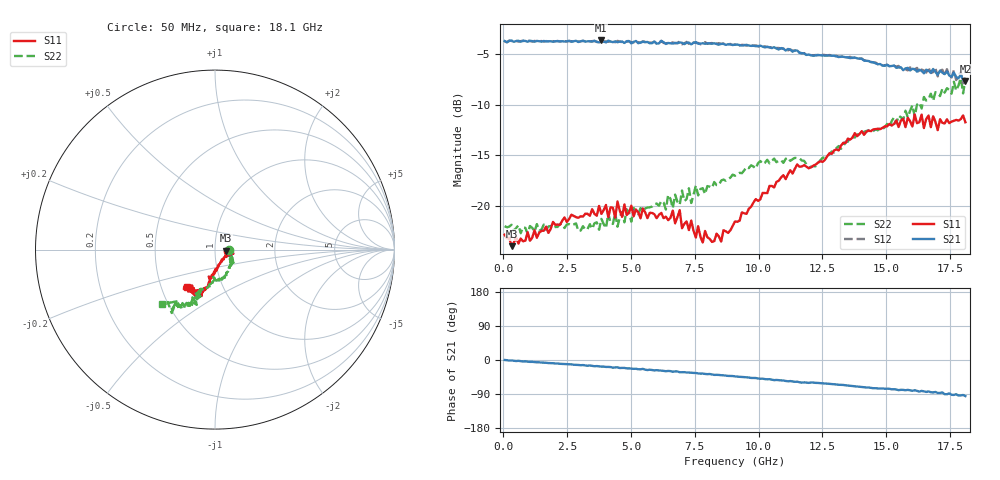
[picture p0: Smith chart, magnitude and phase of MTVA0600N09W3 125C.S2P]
! Network Analyzer HP8720D.06.14 Serial No. US36140669
! 10 May 2005  15:08:20
! Frequency  S11  S21  S12  S22
# HZ  S  DB R 50
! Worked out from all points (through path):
!   201 points, 50 MHz to 18.1 GHz, reference 50 ohm
!   highest |S21| = -3.67 dB at 3.841 GHz (marker M1); lowest = -7.7 dB at 18.1 GHz (marker M2)
!   group delay of S21, straight-line fit = 14.5 ps
!   lowest |S11| = -23.9 dB at 320.8 MHz (marker M3), VSWR 1.14, Z = 56.7 - j0.663 ohm
!   |S11| at or under -10 dB: start of sweep to end of sweep
!   |S22| runs from -22.7 to -7.4 dB; largest |S21 - S12| = 0.028
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5e7  -22.81 -4.4  -3.73 0.1  -3.77 -0.5  -21.97 -3.6
3.2075e8  -23.94 -5.3  -3.67 -1.1  -3.72 -1.3  -21.83 -5.6
3.1185e9  -21.03 -13.8  -3.69 -13.4  -3.73 -13.9  -21.98 -19.0
3.8405e9  -20.76 -8.7  -3.67 -17.4  -3.72 -17.3  -21.25 -23.6
4.382e9  -21.12 -11.7  -3.76 -19.5  -3.85 -20.1  -20.68 -19.0
4.47225e9  -19.54 -12.5  -3.85 -19.3  -3.71 -20.5  -22.02 -16.8
4.65275e9  -21.06 -14.8  -3.77 -20.9  -3.85 -21.8  -20.57 -16.2
4.743e9  -19.83 -9.7  -3.92 -20.9  -3.77 -21.5  -21.59 -20.3
6.09675e9  -20.85 -11.5  -3.96 -27.5  -3.88 -28.2  -19.96 -24.3
6.63825e9  -20.44 -9.4  -3.98 -31.1  -3.86 -31.1  -20.21 -32.4
6.7285e9  -21.70 -7.2  -3.91 -30.0  -3.96 -30.0  -18.87 -33.4
6.909e9  -20.40 -11.5  -3.87 -32.3  -3.78 -32.5  -19.86 -34.5
6.99925e9  -22.18 -13.3  -3.90 -32.3  -4.05 -32.6  -18.46 -32.2
7.36025e9  -21.41 -21.1  -4.05 -33.5  -3.92 -34.7  -19.69 -32.8
7.8115e9  -23.58 -30.6  -3.95 -35.8  -3.98 -36.6  -18.23 -39.8
9.075e9  -21.51 -69.6  -4.09 -43.3  -4.07 -43.9  -17.01 -61.1
1.151175e10  -15.88 -96.9  -4.67 -57.2  -4.60 -58.1  -15.27 -87.5
1.21435e10  -16.00 -99.9  -5.17 -59.5  -5.14 -60.3  -16.07 -91.1
1.512175e10  -11.89 -107.8  -6.21 -75.8  -6.21 -76.9  -12.26 -108.8
1.79195e10  -11.43 -129.7  -7.04 -93.5  -6.80 -91.3  -7.38 -124.3
1.800975e10  -11.06 -128.4  -7.57 -92.3  -7.90 -95.2  -8.89 -126.7
1.81e10  -11.73 -126.9  -7.66 -95.2  -7.33 -96.8  -7.46 -133.9
